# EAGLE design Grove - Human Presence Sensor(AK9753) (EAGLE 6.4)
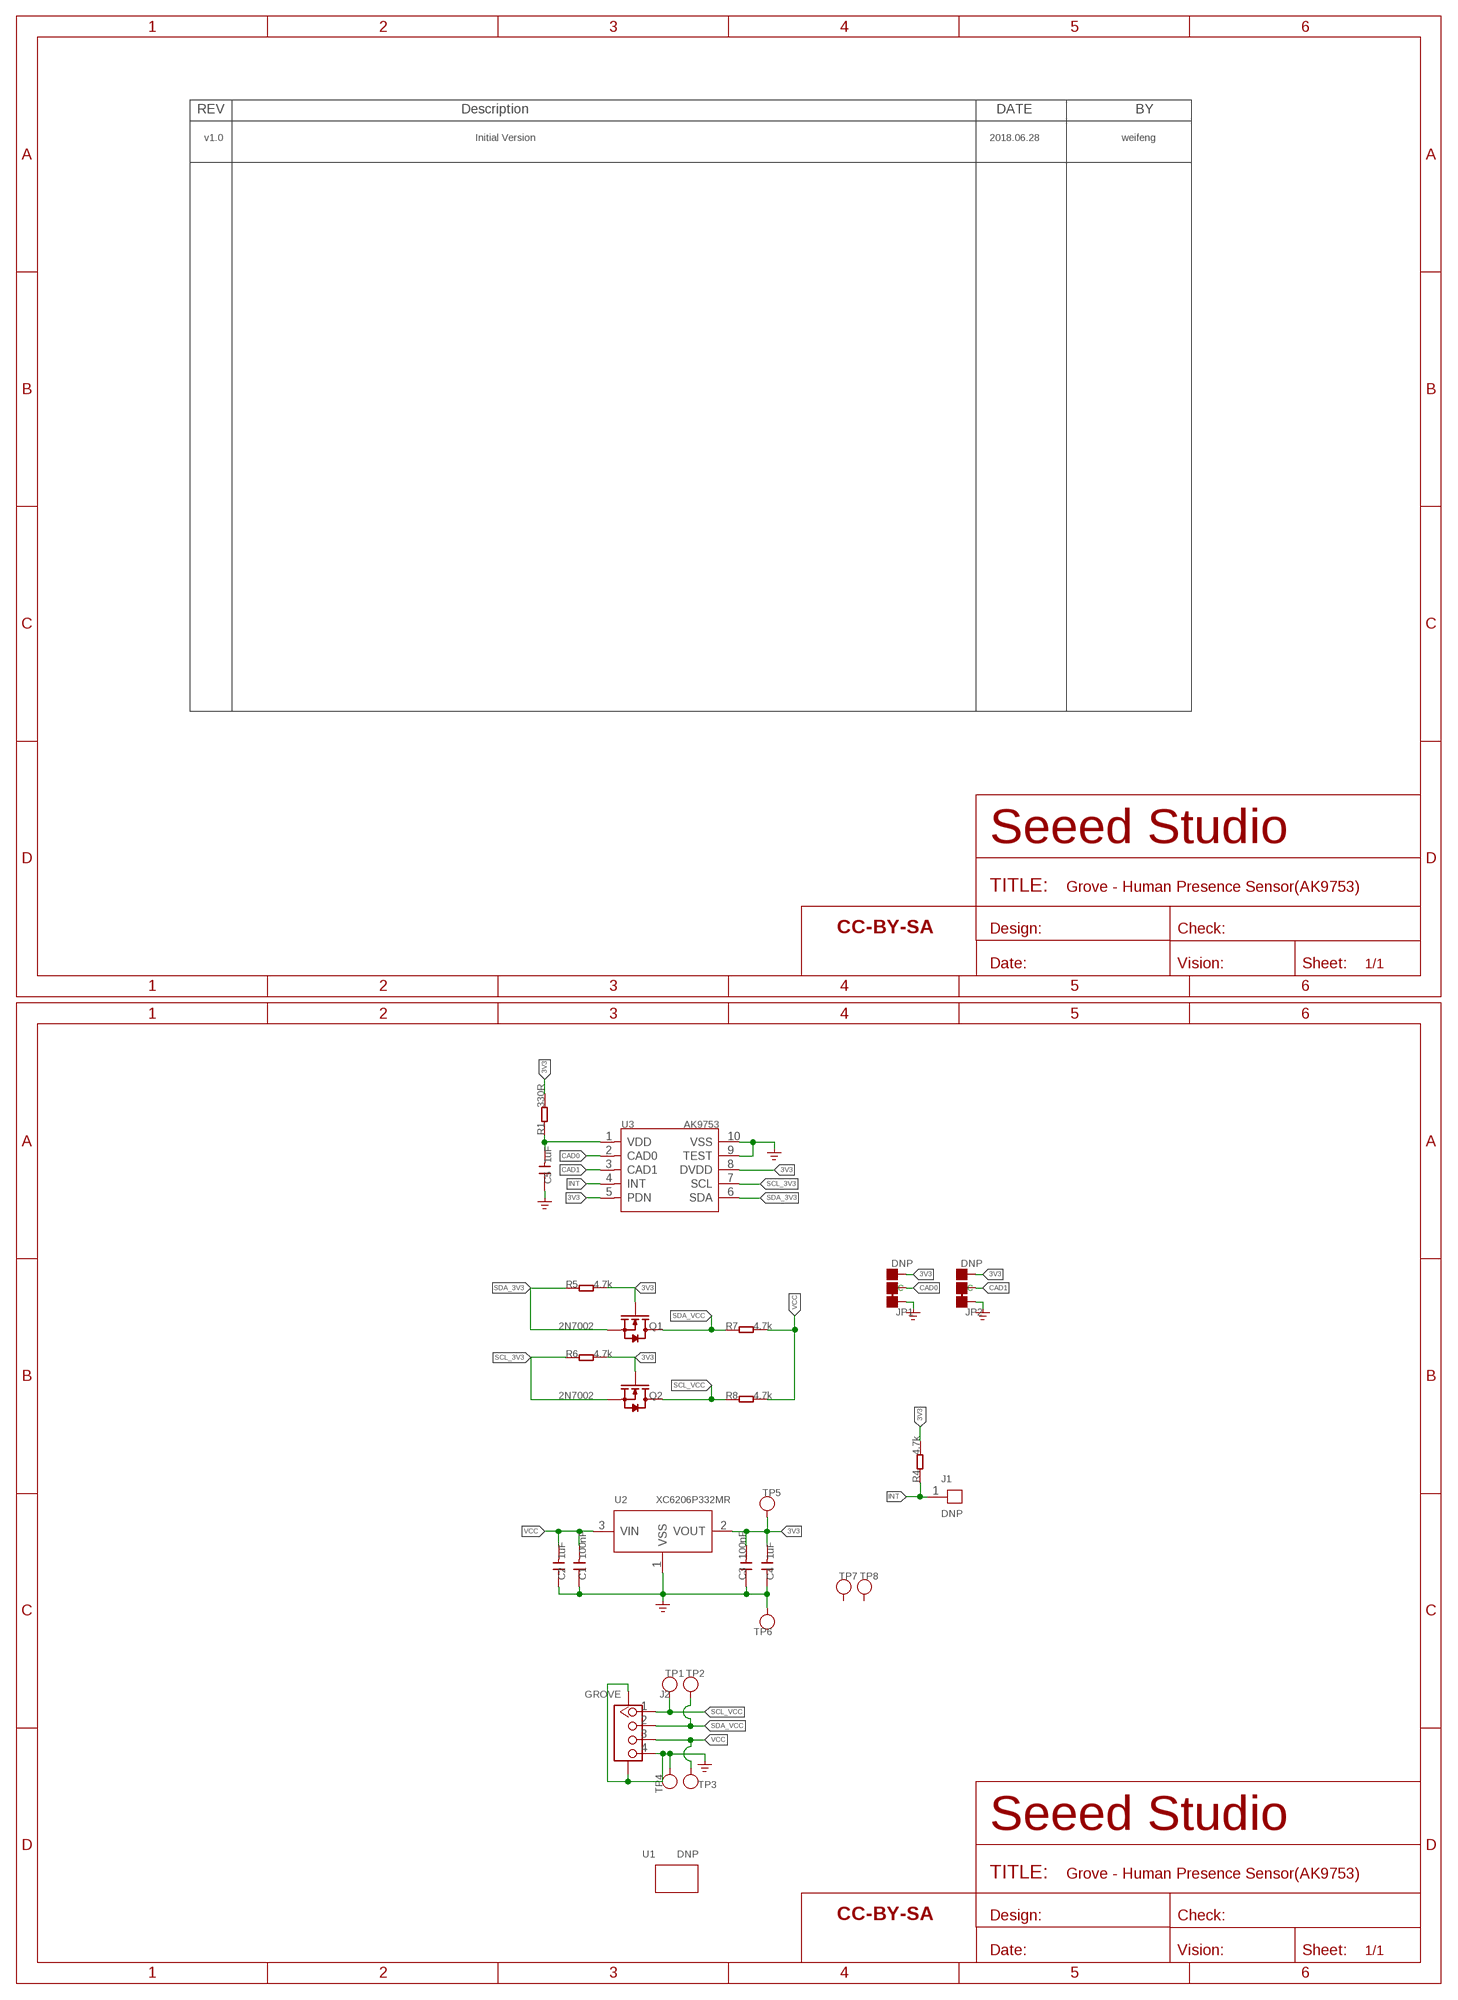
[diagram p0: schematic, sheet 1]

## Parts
C1  100nF  CAP-0603  [C0603]
C2  1uF  CAP-0603  [C0603]
C3  100nF  CAP-0603  [C0603]
C4  1uF  CAP-0603  [C0603]
C5  1uF  CAP-0603  [C0603]
FR1  SEEEDSTUDIO-OPEN-SCH-FRAME  [SEEEDSTUDIO-PCB-FRAME]
J1  DNP  HEADER-1P-35  [1P-65/35MIL]
J2  GROVE  GROVE-CONNECTOR-SMD'90D'  [HW4-SMD-2.0-90D]
JP1  DNP  JP-3P-SHORT  [3P-SMD-SHORT]
JP2  DNP  JP-3P-SHORT  [3P-SMD-SHORT]
Q1  2N7002  MOSFET-N'SOT23'  [SOT-23]
Q2  2N7002  MOSFET-N'SOT23'  [SOT-23]
R1  330R  RES-0603  [R0603]
R4  4.7k  RES-0603  [R0603]
R5  4.7k  RES-0603  [R0603]
R6  4.7k  RES-0603  [R0603]
R7  4.7k  RES-0603  [R0603]
R8  4.7k  RES-0603  [R0603]
TP1  TEST-POINT'4545'  [TP-D45MIL]
TP2  TEST-POINT'4545'  [TP-D45MIL]
TP3  TEST-POINT'4545'  [TP-D45MIL]
TP4  TEST-POINT'4545'  [TP-D45MIL]
TP5  TEST-POINT'4545'  [TP-D45MIL]
TP6  TEST-POINT'4545'  [TP-D45MIL]
TP7  TEST-POINT'4545'  [TP-D45MIL]
TP8  TEST-POINT'4545'  [TP-D45MIL]
U1  DNP  GROVE-BOTTOM  [GROVE-1*2-TEST-PLATFORM-BOTTOM]
U2  XC6206P332MR  PMIC-XC6206PMR  [SOT-23]
U3  AK9753  SENSOR-AK9753  [SON10-0.65-4.6X3.8X0.99MM]
U$4  SEEEDSTUDIO-OPEN-SCH-FRAME  [SEEEDSTUDIO-PCB-FRAME]

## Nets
3V3: C3.2 C4.2 JP1.00(R) JP2.00(R) Q1.1(G) Q2.1(G) R1.2 R4.2 R5.2 R6.2 TP5.T U2.2(VOUT) U3.5(PDN) U3.8(DVDD)
CAD0: JP1.MM(C) U3.2(CAD0)
CAD1: JP2.MM(C) U3.3(CAD1)
GND: C1.1 C2.1 C3.1 C4.1 C5.1 J2.4 J2.SS1 J2.SS2 JP1.11(L) JP2.11(L) TP4.T TP6.T U2.1(VSS) U3.9(TEST) U3.10(VSS) ; supply symbol labelled GND_POWER
INT: J1.1 R4.1 U3.4(INT)
N$2: C5.2 R1.1 U3.1(VDD)
SCL_3V3: Q2.2(S) R6.1 U3.7(SCL)
SCL_VCC: J2.1 Q2.3(D) R8.1 TP1.T
SDA_3V3: Q1.2(S) R5.1 U3.6(SDA)
SDA_VCC: J2.2 Q1.3(D) R7.1 TP2.T
VCC: C1.2 C2.2 J2.3 R7.2 R8.2 TP3.T U2.3(VIN)
Unconnected: TP7.T TP8.T

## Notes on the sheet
- v1.0 | Initial Version | 2018.06.28 | weifeng

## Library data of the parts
C1-C5 = Discrete-new:CAP: Ceramic Capacitors
FR1 U$4 = moudle-new:SEEEDSTUDIO-OPEN-SCH-FRAME
J1 = Connector-new:HEADER-1P
J2 = Connector-new:GROVE-CONNECTOR-SMD: 4P-SMD-2.0:320110030;4P-SMD-2.0-90D:320110032
JP1 JP2 = Discrete-new:JP-3P-SHORT
Q1 Q2 = Discrete-new:MOSFET-N
R1 R4-R8 = Discrete-new:RES
TP1-TP8 = Discrete-new:TEST-POINT; PARTNO: DNP
U1 = moudle-new:GROVE
U2 = IC-new:PMIC-XC6206P: LOW ESR Cap.Compatible Positive Voltage Regulators
U3 = Discrete-new:SENSOR-AK9753; PROD_ID: SEN-13737; VALUE: AK9750

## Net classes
3 usbvcc: width 0.203 mm, drill 0.305 mm, clearance 0.203 mm

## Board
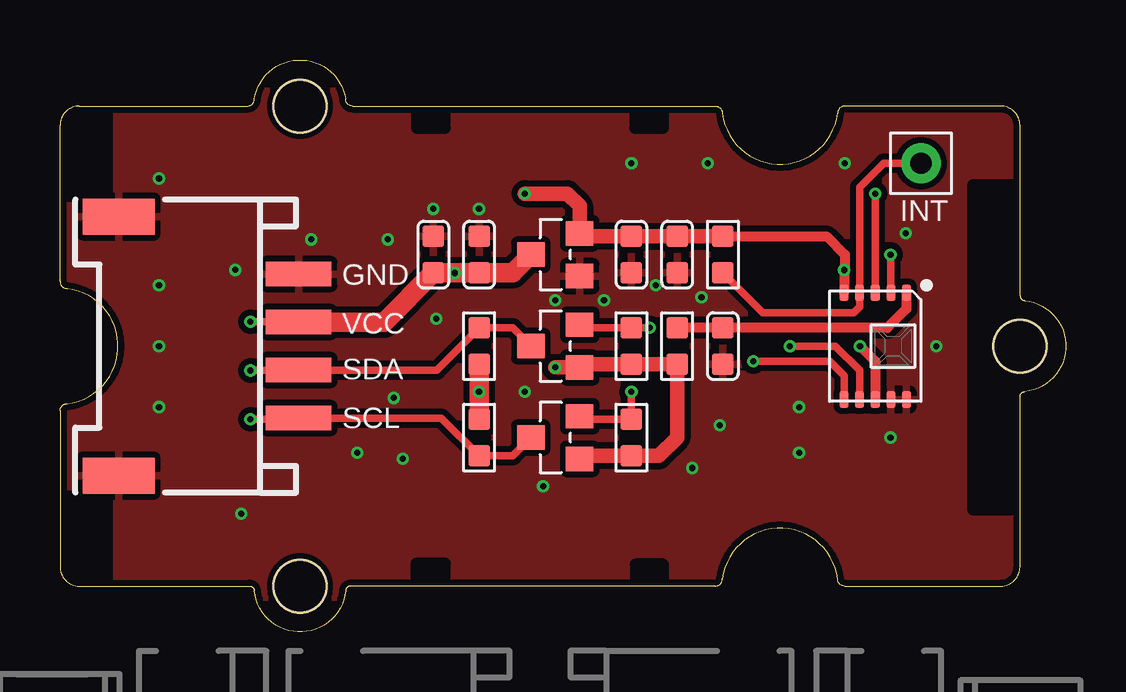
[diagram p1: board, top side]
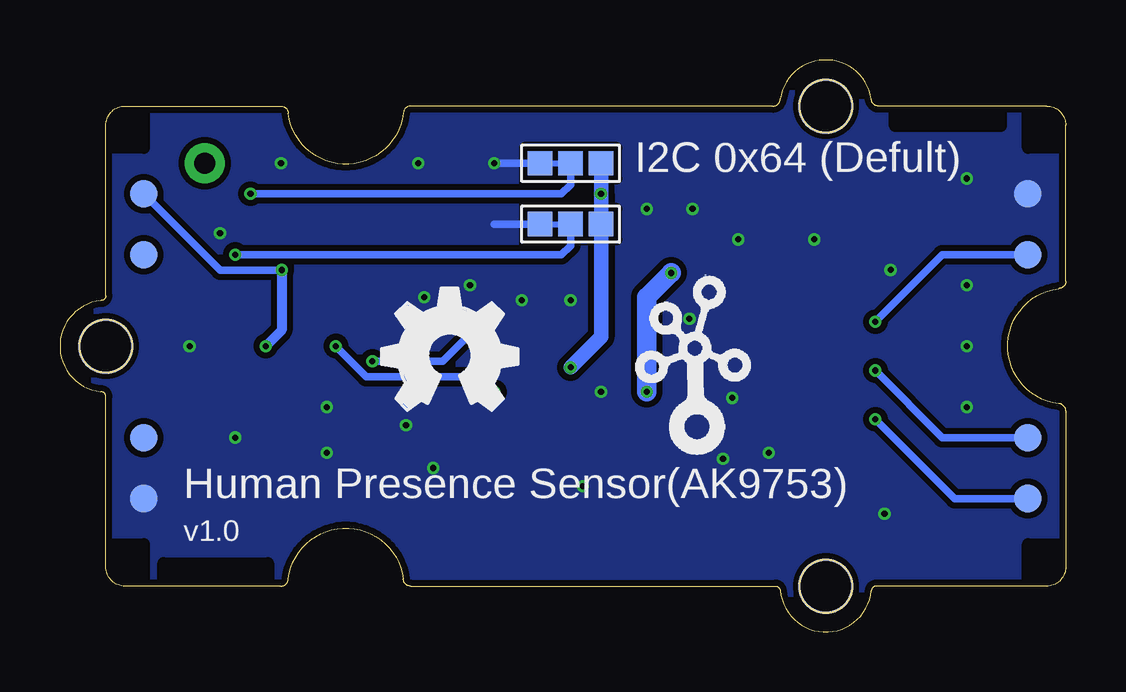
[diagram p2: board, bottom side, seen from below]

Size 41.91 x 23.83 mm. Coordinates in mm from the lower left corner, seen from the top.
Copper layers (1*16): Top 0.035mm / dielectric 1.5mm / Bottom 0.035mm
Design rules "SeeedStudio_2layer_DRU_no_angle_20140221": minimum track width 1mil, minimum drill 10mil, track to track 6mil, track to pad 6mil, pad to pad 6mil, via to via 6mil, smd to smd 0mil, copper to edge 10mil, drill to drill 10mil, minimum pad ring 4mil, minimum via ring 4mil, stop-mask expansion 2mil, vias tented up to drill 25mil, thermal gap 10mil

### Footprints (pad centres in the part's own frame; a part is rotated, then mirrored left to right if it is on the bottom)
C0603 = smd 0.889 x 0.889: 1 0,0.762; 2 0,-0.762
1P-65/35MIL = drill 0.889 pad 1.651: 1 0,0
HW4-SMD-2.0-90D = smd 1.01 x 2.74: 1 -3,-0.1; 2 -1,-0.1; 3 1,-0.1; 4 3,-0.1 | smd 1.5 x 3: SS1 -5.4,7.4; SS2 5.4,7.4
3P-SMD-SHORT = smd 1.016 x 1.016: 00 -1.27,0; 11 1.27,0; MM 0,0
SOT-23 = smd 1.143 x 1.016: 1 1.016,-0.889; 2 1.016,0.889; 3 -1.016,0
R0603 = smd 0.889 x 0.889: 1 0,0.762; 2 0,-0.762
TP-D45MIL = smd 1.143 x 1.143: T 0,0
GROVE-1*2-TEST-PLATFORM-BOTTOM = hole 2.2: 10.635,10; 10.635,-10; -19.365,0
SOT-23' = smd 1.016 x 1.143: 1 -0.889,-1.016; 2 0.889,-1.016; 3 0,1.016
SON10-0.65-4.6X3.8X0.99MM = smd 0.7 x 0.38: 1 -2.225,1.3; 2 -2.225,0.65; 3 -2.225,0; 4 -2.225,-0.65; 5 -2.225,-1.3; 6 2.225,-1.3; 7 2.225,-0.65; 8 2.225,0; 9 2.225,0.65; 10 2.225,1.3

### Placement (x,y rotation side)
C1  17.46,15.72 0 top
C2  15.56,15.72 0 top
C3  25.72,15.72 180 top
C4  23.81,15.72 180 top
C5  27.62,11.91 180 top
FR1  not placed on the board
J1  35.88,19.53 0 top
J2  9.84,11.91 90 top
JP1  20.64,16.99 180 bottom
JP2  20.64,19.53 180 bottom
Q1  20.64,11.91 0 top
Q2  20.64,8.1 0 top
R1  25.72,11.91 0 top
R4  27.62,15.72 180 top
R5  23.81,11.91 0 top
R6  23.81,8.1 0 top
R7  17.46,11.91 0 top
R8  17.46,8.1 180 top
TP1  1.59,5.56 0 bottom
TP2  1.59,8.1 0 bottom
TP3  1.59,15.72 0 bottom
TP4  1.59,18.26 0 bottom
TP5  38.42,18.26 180 bottom
TP6  38.42,5.56 180 bottom
TP7  38.42,8.1 180 bottom
TP8  38.42,15.72 180 bottom
U1  20.64,11.91 180 top
U2  XC6206P332MR  [SOT-23']  20.64,15.72 90 top
U3  33.97,11.91 270 top
U$4  not placed on the board
U$9  [TWIGLOGO]  15.43,8.35 0 bottom
U$10  [OSHW_FILLX200_NOTEXT]  28.51,9.24 0 bottom

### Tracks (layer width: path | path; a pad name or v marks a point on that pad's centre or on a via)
3V3  (via drill 0.25 pad 0.51)
  Top 0.406: R4.2 31.94,16.48 32.7,15.72 32.7,15.11 v32.67,15.08 U3.5 | v33.34,11.91 33.97,11.27 U3.8
  Top 0.61: R4.2 C3.2 C4.2 21.78,16.48 U2.2 21.65,17.75 21.14,18.26 v19.37,18.26 | Q2.1 21.78,7.34 R6.2 24.95,7.34 25.72,8.1 R1.2 R5.2 21.78,11.15 Q1.1 v20.64,11.02
  Bottom 0.305: v32.67,15.08 35.23,15.08 TP5.T
  Bottom 0.406: v32.67,15.08 32.67,12.57 v33.34,11.91
  Bottom 0.61: v20.64,11.02 19.37,12.29 JP1.00 v19.37,18.26 JP2.00
CAD0  (via drill 0.25 pad 0.51)
  Top 0.305: v34.61,15.72 34.61,14.15 U3.2
  Bottom 0.305: JP1.MM 20.64,16.1 21.02,15.72 v34.61,15.72
CAD1  (via drill 0.25 pad 0.51)
  Top 0.305: U3.3 v33.97,18.26
  Bottom 0.305: JP2.MM 20.64,18.64 21.02,18.26 v33.97,18.26
GND  (via drill 0.25 pad 0.51)
  Bottom 0.305: JP1.11 23.81,16.99 | JP2.11 v23.81,19.53
  other vias: 7.3,15.08 4.12,11.91 7.55,4.92 4.12,9.37 4.12,14.45 15.56,17.62 17.46,17.62 20.64,13.81 30.8,9.37 15.68,13.05 13.9,9.75 4.12,18.89 13.65,16.35 10.48,16.35 19.37,10 14.29,7.21 12.38,7.46 22.67,13.81 24.83,14.45 26.73,13.94 27.49,8.61 34.61,8.1 36.51,11.91 26.98,19.53 32.7,19.53 35.24,16.61 26.35,6.83 20.13,6.07 30.8,7.46
  pour Bottom (isolate 0.254): -0.32,23.97 42.23,23.97 42.23,-0.16 -0.32,-0.16
  pour Top (isolate 0.254): -0.32,23.97 42.23,23.97 42.23,-0.16 -0.32,-0.16
INT
  Top 0.305: J1.1 34.32,19.53 33.32,18.53 U3.4 33.32,13.54 33.08,13.31 29.27,13.31 R4.1
N$2
  Top 0.406: U3.1 35.27,13.46 34.48,12.67 C5.2 R1.1
SCL_3V3  (via drill 0.25 pad 0.51)
  Top 0.305: Q2.2 21.78,8.86 R6.1 v23.81,10 | U3.7 33.32,10.9 32.31,11.91 v30.41,11.91
  Bottom 0.305: v23.81,10 24.45,10.64 29.14,10.64 v30.41,11.91
SCL_VCC  (via drill 0.25 pad 0.51)
  Top 0.305: Q2.3 18.86,7.34 R8.1 15.89,8.91 J2.1 9.89,8.86 v7.94,8.86
  Bottom 0.305: TP1.T 4.63,5.56 v7.94,8.86
SDA_3V3  (via drill 0.25 pad 0.51)
  Top 0.305: Q1.2 21.78,12.67 R5.1 v24.57,12.67 | U3.6 32.67,10.67 32.06,11.27 v28.89,11.27
  Bottom 0.305: v28.89,11.27 25.97,11.27 v24.57,12.67
SDA_VCC  (via drill 0.25 pad 0.51)
  Top 0.305: Q1.3 18.86,12.67 R7.1 15.7,10.91 J2.2 9.92,10.89 v7.94,10.89
  Bottom 0.305: TP2.T 5.14,8.1 v7.94,10.89
VCC  (via drill 0.25 pad 0.51)
  Top 0.305: v7.94,12.92 9.92,12.92 J2.3
  Top 0.813: J2.3 13.51,12.91 C2.2 v16.44,14.96 C1.2 17.97,14.96 18.86,14.96 U2.3 | R8.2 v17.46,10 R7.2
  Bottom 0.305: TP3.T 5.14,15.72 v7.94,12.92
  Bottom 0.813: v17.46,10 17.46,13.94 v16.44,14.96

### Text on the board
tPlace: INT
bPlace: I2C 0x64 (Defult) | Human Presence Sensor(AK9753) | v1.0
tNames: GND | VCC | SDA | SCL

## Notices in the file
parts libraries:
moudle-new: This work is licensed under the Creative Commons Attribution 4.0 International License.
To view a copy of this license,visit:
http://creativecommons.org/licenses/by-sa/4.0
moudle-new: CC-BY-SA
